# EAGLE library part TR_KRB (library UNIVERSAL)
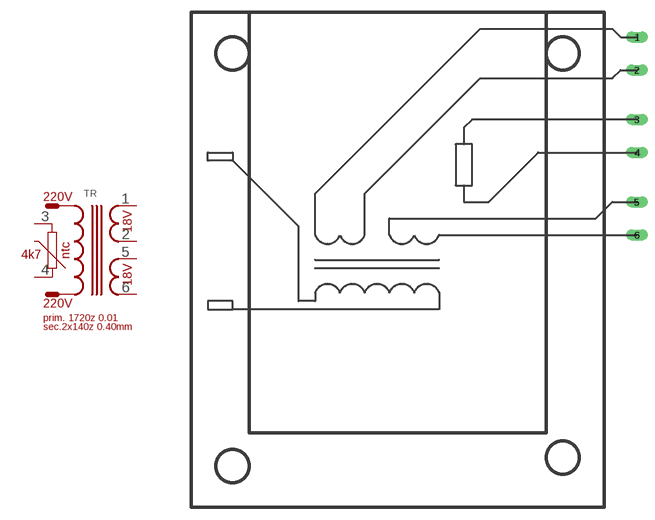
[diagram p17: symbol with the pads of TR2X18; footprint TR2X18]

Designator prefix TR

## TR_KRB  [TR2X18]
1  1
2  2
3  3
4  4
5  5
6  6

## Footprint TR2X18 (pad centres in mm)
drill 0.813 pad 1.27 long: 1 54,57; 2 54,53; 3 54,47; 4 54,43; 5 54,37; 6 54,33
